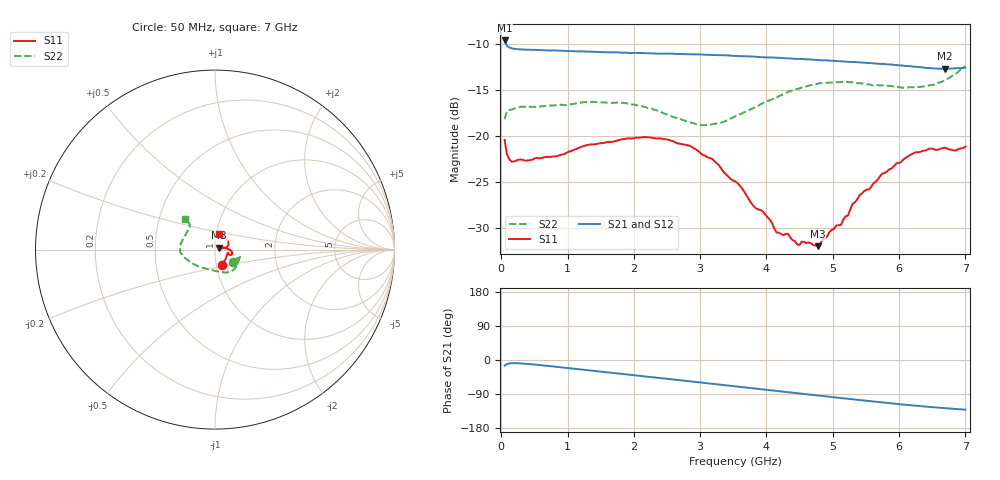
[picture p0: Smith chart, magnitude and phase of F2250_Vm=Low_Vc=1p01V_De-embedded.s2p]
! Integrated Device Technology
! Corporate Headquarters
! 6024 Silver Creek Valley Road
! San Jose, CA 95138  USA
! Phone:  1-408-284-8200
! Toll Free:  1-800-223-1366
! Webpage:  http://www.idt.com/
! Timing and RF Division
! 515 Groton Road, Suite 102
! Westford, MA 01886-6024
! Device:  F2250
! Description: Voltage Variable RF Attenuator
! Frequency:  50.0 -  6000.00 MHz
! Package:  3x3 mm Thin QFN Plastic Package: 16 pin
! Ports:  2 RF, 3 DC
!  Pin  1  = GND
!  Pin  2  = NC
!  Pin  3  = RF1  = Port 1
!  Pin  4  = NC
!  Pin  5  = GND
!  Pin  6  = GND
!  Pin  7  = GND
!  Pin  8  = GND
!  Pin  9  = NC
!  Pin 10  = RF2  = Port 2
!  Pin 11  = NC
!  Pin 12  = GND
!  Pin 13  = GND
!  Pin 14  = VCNTRL
!  Pin 15  = VDD
!  Pin 16  = VMODE
! Vcntrl:  1.010 Volts
! Vmode:  +0.000 Volts
! Vdd:  +3.30  Volts
! Current:  1.187 mA
! Data:  The device was measured on a the F2250 evaluation board which has
!  individual transmission lines to the RF pins.  Data was collected
!  using a calibrated network analyzer.  The evaluation board was
!  de-embedded using a TRL calibration technique.
!  The reference plane is the edge of the package pin.
! Misc:  SN 10
!  Action Tracker AT0258
! Date Measured:  2014-11-26
! Date:  2015-10-15  MJV
! Note:
!  Integrated Device Technology supplies this data as a sample of measured
!  data at the package pin for this product.  Your particular data for this
!  product may vary.
!  Data was taken at 25 degrees C.
!  Integrated Device Technology reserves the right to change this data at anytime.
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# GHz S dB R 50
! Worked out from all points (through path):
!   201 points, 50 MHz to 7 GHz, reference 50 ohm
!   highest |S21| = -9.61 dB at 50 MHz (marker M1); lowest = -12.7 dB at 6.687 GHz (marker M2)
!   group delay of S21, straight-line fit = 52.1 ps
!   lowest |S11| = -32.0 dB at 4.776 GHz (marker M3), VSWR 1.05, Z = 52.4 + j1.05 ohm
!   |S11| at or under -10 dB: start of sweep to end of sweep
!   |S22| runs from -18.8 to -12.4 dB; largest |S21 - S12| = 0.00082
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0.05  -20.42 -67.6  -9.61 -15.0  -9.61 -15.0  -18.16 -34.4
0.08475  -21.97 -42.0  -10.19 -10.8  -10.18 -10.7  -17.29 -19.0
0.15425  -22.78 -25.8  -10.46 -8.5  -10.46 -8.5  -17.12 -13.5
0.84925  -22.17 -16.9  -10.72 -18.3  -10.71 -18.3  -16.63 -30.7
1.2315  -21.11 -19.5  -10.80 -25.5  -10.81 -25.5  -16.32 -41.3
1.857  -20.33 -16.3  -10.94 -37.2  -10.94 -37.2  -16.40 -55.0
2.37825  -20.25 -10.5  -11.03 -47.1  -11.03 -47.1  -17.28 -68.3
3.0385  -22.04 -0.2  -11.15 -60.0  -11.15 -60.0  -18.83 -100.3
3.525  -24.92 8.0  -11.28 -69.5  -11.28 -69.5  -17.86 -130.7
3.803  -27.60 14.8  -11.35 -75.0  -11.35 -75.0  -16.95 -144.5
4.04625  -29.06 22.1  -11.46 -79.7  -11.45 -79.7  -16.11 -155.1
4.1505  -30.47 24.2  -11.49 -81.7  -11.49 -81.7  -15.79 -159.0
4.32425  -30.64 25.0  -11.56 -85.0  -11.56 -85.0  -15.21 -164.2
4.46325  -31.79 27.4  -11.61 -87.8  -11.60 -87.8  -14.88 -168.0
4.7065  -31.89 26.9  -11.71 -92.4  -11.71 -92.5  -14.44 -173.8
4.776  -31.98 23.5  -11.73 -93.8  -11.73 -93.8  -14.29 -175.3
5.1235  -29.66 14.2  -11.87 -100.4  -11.88 -100.4  -14.14 177.0
5.4015  -26.45 10.1  -11.99 -105.6  -11.99 -105.7  -14.27 170.5
5.85325  -23.62 11.9  -12.22 -113.9  -12.20 -114.0  -14.57 159.0
6.2355  -21.80 21.7  -12.46 -120.5  -12.45 -120.6  -14.71 146.4
6.68725  -21.26 45.4  -12.69 -126.8  -12.68 -126.9  -13.89 134.8
7  -21.15 75.5  -12.58 -131.2  -12.58 -131.2  -12.37 134.8
